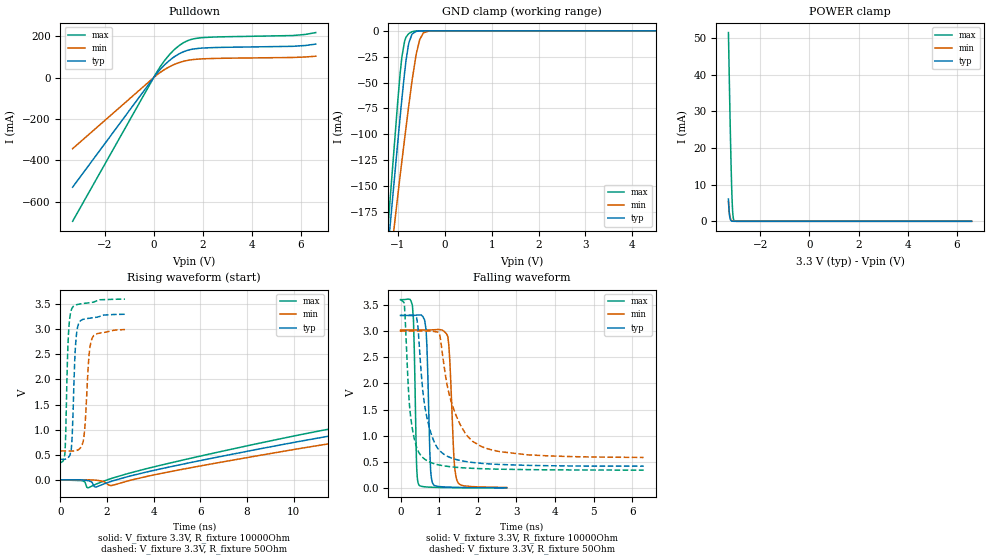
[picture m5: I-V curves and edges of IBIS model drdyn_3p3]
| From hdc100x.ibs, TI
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|   drdyn_3p3 Model
[Model]   drdyn_3p3
Model_type   Open_drain
Polarity   Non-Inverting
Vmeas = 1.65
Vref = 3.3
Cref = 2pF
Rref = 10000
|   typ   min   max
|   (nom PVT)   (fast PVT)   (slow PVT)
C_comp   2.652e-12   2.599e-12   2.690e-12
| Where nom  PVT is Nominal Process, 3.3V, 27C
|   Fast PVT is Strong Process,  3.6V, -40C
|   Slow PVT is Weak Process,   3V, 150C
[Voltage Range]   3.3   3   3.6
|Junction Temperature
[Temperature Range]   27   150   -40
[Pullup Reference]   3.3   3   3.6
[Pulldown Reference]   0   0   0
[Power Clamp Reference]   3.3   3   3.6
[GND Clamp Reference]   0   0   0
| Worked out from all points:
|   slope of the pulldown table from 0 to 0.495 V, typ, clamps not added: 7.34 ohm
|   GND clamp passes 1 mA (typ) near -0.62 V on its own axis
|   POWER clamp passes 1 mA (typ) near -3.24 V on its own axis
|   falling waveform, V_fixture 3.3V, R_fixture 10000Ohm: 20-80 % time 73.5ps typ, 103ps min, 59ps max; typ from 3.3 V to 0.005 V
|   rising waveform, V_fixture 3.3V, R_fixture 10000Ohm: 20-80 % time 28.2ns typ, 29.2ns min, 27.8ns max; typ from 0.002 V to 3.29 V
|   falling waveform, V_fixture 3.3V, R_fixture 50Ohm: 20-80 % time 326ps typ, 566ps min, 203ps max; typ from 3.3 V to 0.418 V
|   rising waveform, V_fixture 3.3V, R_fixture 50Ohm: 20-80 % time 142ps typ, 185ps min, 121ps max; typ from 0.413 V to 3.3 V
[Pulldown]
|   Voltage   I(typ)   I(min)   I(max)
-3.3V     -529mA     -342.9mA   -693.7mA
134.4mV   21.17mA    13.45mA    28.23mA
432mV     60.41mA    38.38mA    80.64mA
652.8mV   84.1mA     53.37mA    112.6mA
1.031V    114.6mA    72.51mA    154.3mA
1.442V    134.1mA    84.69mA    181.3mA
1.905V    142.3mA    90.36mA    192.5mA
5.655V    151.4mA    97.44mA    203.4mA
6.6V      162mA      103.5mA    217.8mA
[GND Clamp]
|   Voltage   I(typ)   I(min)   I(max)
-3.3V     -1.065A    -981.6mA   -1.128A
-1.381V   -296.4mA   -310.1mA   -290.7mA
-1.007V   -111.2mA   -162.5mA   -72.07mA
-913.2mV  -66.43mA   -126.5mA   -25.75mA
-852mV    -39.52mA   -103.9mA   -9.654mA
-776.4mV  -14.76mA   -76.41mA   -3.217mA
-699mV    -3.566mA   -49.58mA   -930.7uA
-609mV    -572.4uA   -23.07mA   -104.1uA
-534mV    -101.3uA   -8.763mA   -10.44uA
-453mV    -12.35uA   -1.908mA   -596.2nA
-330mV    -322nA     -97.29uA   0A
6.6V      0A         0A         0A
[POWER Clamp]
|   Voltage   I(typ)   I(min)   I(max)
-3.3V     6.079mA    5.422mA    51.48mA
-3.285V   4.075mA    3.945mA    45.96mA
-3.26V    1.908mA    2.239mA    37.15mA
-3.237V   849uA      1.253mA    29.12mA
-3.216V   393.1uA    727.4uA    22.33mA
-3.185V   120.4uA    316.3uA    13.31mA
-3.163V   52.62uA    175.5uA    8.179mA
-3.142V   22.84uA    96.55uA    4.338mA
-3.12V    9.942uA    52.54uA    1.948mA
-3.098V   4.309uA    28.13uA    761.6uA
-3.052V   706.8nA    6.22uA     80.17uA
6.6V      0A         0A         0A
[Ramp]
R_load = 10000
|   typ   min   max
dV/dt_r   1.97828/2.82675e-08   1.81076/2.92693e-08   2.15862/2.78207e-08
dV/dt_f   1.97877/7.36257e-11   1.81141/1.0434e-10   2.15899/5.90513e-11
[Falling Waveform]
V_fixture = 3.3V
V_fixture_min = 3V
V_fixture_max = 3.6V
R_fixture = 10000Ohm
|   Time   V(typ)   V(min)   V(max)
0s        3.3V       3V         3.6V
307.1ps   3.301V     3.022V     3.493V
413.9ps   3.306V     3.022V     483.1mV
475.3ps   3.309V     3.022V     60.04mV
660.2ps   3.034V     3.022V     21.24mV
758.3ps   682.3mV    3.023V     16.88mV
836.1ps   82.22mV    3.025V     14.4mV
1.228ns   17.69mV    2.874V     7.938mV
1.479ns   12.16mV    115.1mV    6.222mV
2.745ns   4.67mV     10.29mV    3.31mV
[Rising Waveform]
V_fixture = 3.3V
V_fixture_min = 3V
V_fixture_max = 3.6V
R_fixture = 10000Ohm
|   Time   V(typ)   V(min)   V(max)
0s        2.049mV    2.948mV    1.682mV
1.184ns   -13.88mV   3.271mV    -156.4mV
1.51ns    -140.4mV   -3.47mV    -86.43mV
2.181ns   -26.92mV   -111mV     30.01mV
13.79ns   1.058V     890.2mV    1.216V
31.29ns   2.131V     1.892V     2.375V
38.03ns   2.717V     2.31V      3.077V
43.41ns   3.063V     2.691V     3.403V
56.03ns   3.264V     2.967V     3.574V
96.93ns   3.295V     3.014V     3.596V
[Falling Waveform]
V_fixture = 3.3V
V_fixture_min = 3V
V_fixture_max = 3.6V
R_fixture = 50Ohm
|   Time   V(typ)   V(min)   V(max)
0s        3.3V       3V         3.6V
100.7ps   3.3V       3V         3.489V
230.6ps   3.302V     3V         1.595V
417.8ps   3.257V     3V         776.8mV
622.6ps   1.582V     3.001V     553.5mV
1.014ns   712.7mV    2.922V     438.6mV
1.193ns   614.7mV    2.021V     416.3mV
1.399ns   553.8mV    1.46V      399.2mV
2.08ns    473.1mV    798.1mV    370.2mV
6.29ns    417.9mV    584.2mV    342.3mV
[Rising Waveform]
V_fixture = 3.3V
V_fixture_min = 3V
V_fixture_max = 3.6V
R_fixture = 50Ohm
|   Time   V(typ)   V(min)   V(max)
0s        412.8mV    578.3mV    341mV
196.1ps   413.6mV    578.4mV    566.3mV
328.6ps   441.6mV    578.1mV    2.755V
464.4ps   613.3mV    576.8mV    3.38V
637.7ps   2.615V     580.9mV    3.478V
780.1ps   3.113V     606.3mV    3.496V
998.3ps   3.198V     829.3mV    3.512V
1.226ns   3.217V     2.483V     3.525V
1.363ns   3.225V     2.827V     3.534V
2.765ns   3.297V     2.993V     3.598V
